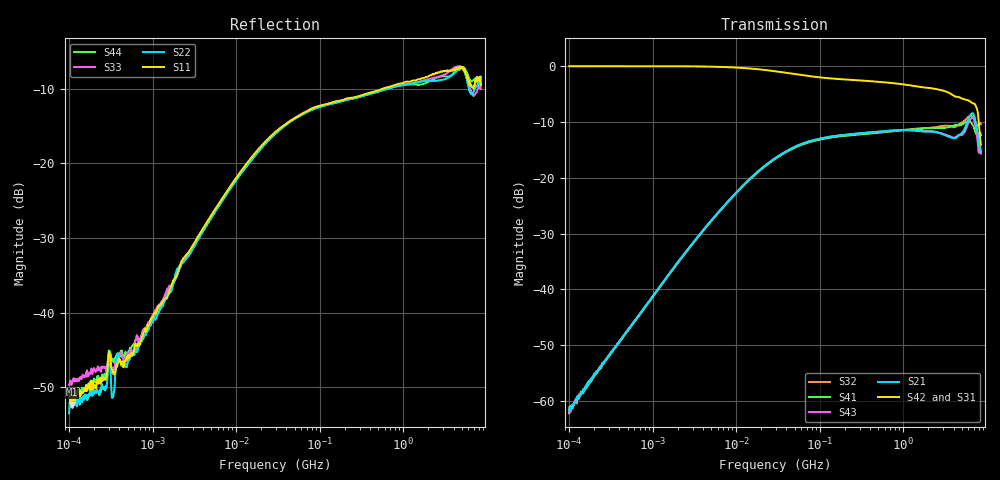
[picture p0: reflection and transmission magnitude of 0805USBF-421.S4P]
# Hz S dB R 50
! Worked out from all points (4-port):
!   801 points, 100 kHz to 8.5 GHz, reference 50 ohm
!   strongest paths, dB at 100 kHz, 1.721 MHz, 29.51 MHz, 502.3 MHz, 8.5 GHz:
!     S42: 0.0, 0.0, -0.9, -2.8, -14.1
!     S31: 0.0, 0.0, -1.0, -2.9, -13.3
!     S21: -61.5, -36.4, -16.5, -11.7, -15.3
!     S43: -61.9, -36.5, -16.5, -11.8, -15.7
!     S41: -62.1, -36.5, -16.6, -11.9, -12.4
!     S32: -62.2, -36.5, -16.6, -12.0, -10.4
!   lowest |S11| = -52.3 dB at 108.3 kHz (marker M1), VSWR 1.00, Z = 50.1 + j0.229 ohm
!   |S11| at or under -10 dB: start of sweep to 573 MHz
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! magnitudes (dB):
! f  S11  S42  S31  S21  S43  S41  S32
! 100 kHz  -50.9  0.0  0.0  -61.5  -61.9  -62.1  -62.2
! 108.3 kHz  -52.3  0.0  0.0  -61.3  -60.9  -60.9  -60.7
! 337.1 kHz  -48.1  0.0  0.0  -50.7  -50.9  -50.9  -50.9
! 34.08 MHz  -15.2  -1.1  -1.1  -15.8  -15.9  -16.0  -16.0
! 3.116 GHz  -7.7  -4.5  -5.0  -12.3  -12.2  -11.1  -10.7
! 6.739 GHz  -9.9  -6.6  -6.8  -8.4  -9.2  -10.5  -9.0
! 8.5 GHz  -9.5  -14.1  -13.3  -15.3  -15.7  -12.4  -10.4
